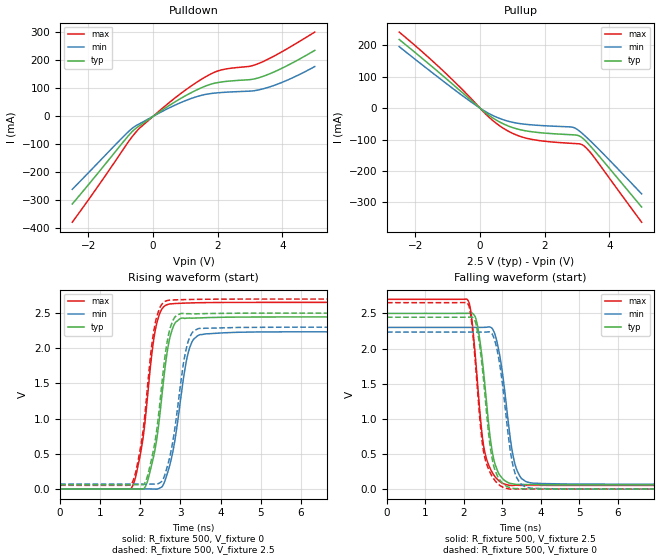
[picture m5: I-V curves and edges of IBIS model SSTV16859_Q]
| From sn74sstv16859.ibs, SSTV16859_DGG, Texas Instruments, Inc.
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[Model]   SSTV16859_Q
Model_type  Output
Vref =   1.25
Rref =   50
Cref =   30p
Vmeas =   1.25
| variable   typ   min   max
C_comp   5.86pF   1.92pF   9.72pF
| C_pullup   7.12pF   1.92pF   9.72pF
| C_pulldown   4.59pF   2.89pF   7.94pF
[Temperature Range]   40   85   0
| Ambient temperature   25   70   0
[Voltage range]   2.5   2.3   2.7
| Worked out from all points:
|   slope of the pulldown table from 0 to 0.375 V, typ, clamps not added: 12.7 ohm
|   slope of the pullup table from 0 to 0.375 V, typ, clamps not added: 12.6 ohm
|   rising waveform, R_fixture 500, V_fixture 0: 20-80 % time 331ps typ, 358ps min, 321ps max; typ from 0 V to 2.44 V
|   falling waveform, R_fixture 500, V_fixture 2.5: 20-80 % time 293ps typ, 319ps min, 272ps max; typ from 2.5 V to 0.06 V
|   rising waveform, R_fixture 500, V_fixture 2.5: 20-80 % time 320ps typ, 340ps min, 313ps max; typ from 0.06 V to 2.5 V
|   falling waveform, R_fixture 500, V_fixture 0: 20-80 % time 286ps typ, 308ps min, 265ps max; typ from 2.44 V to 0 V
[Pulldown]
| SSTV16859_Q
|   Voltage   I(typ)   I(min)   I(max)
-2.5V     -313.2mA   -260.7mA   -378.3mA
-910mV    -89.51mA   -71.28mA   -115.6mA
-550mV    -44.37mA   -34.85mA   -58.82mA
-360mV    -28.68mA   -22.72mA   -36.14mA
700mV     53.31mA    41.25mA    67.71mA
1.38V     96.13mA    71.48mA    124.1mA
1.92V     119mA      83.27mA    158.7mA
2.28V     125.2mA    86.44mA    169.8mA
3.02V     131.7mA    90.39mA    179.8mA
3.44V     144.6mA    99.57mA    197.8mA
4.14V     180.8mA    128.9mA    241.2mA
5V        235.7mA    177.9mA    301.2mA
[Pullup]
| SSTV16859_Q
|   Voltage   I(typ)   I(min)   I(max)
-2.5V     218.3mA    195.6mA    241.8mA
-1.265V   113.1mA    95.84mA    130.6mA
-165mV    15.03mA    11.66mA    18.54mA
305mV     -24.89mA   -18.76mA   -31.42mA
750mV     -51.43mA   -38.03mA   -65.87mA
1.13V     -65.79mA   -47.58mA   -85.66mA
1.525V    -74.13mA   -52.67mA   -97.93mA
2.85V     -84.82mA   -60.61mA   -112.3mA
3.055V    -87.94mA   -71.4mA    -113.6mA
3.22V     -99.68mA   -85.74mA   -120.6mA
3.51V     -132mA     -114mA     -153.5mA
5V        -314.6mA   -273mA     -363mA
[Ramp]
| SSTV16859_Q
| variable   typ   min   max
dV/dt_r   1.47/3.32E-10   1.34/3.64E-10   1.59/3.26E-10
dV/dt_f   1.47/2.94E-10   1.34/3.25E-10   1.59/2.77E-10
R_load = 500
[Rising Waveform]
| SSTV16859_Q
R_fixture =   500
C_fixture =   0
L_fixture =   0
V_fixture =   0
V_fixture_min = 0
V_fixture_max = 0
|   Time   V(typ)   V(min)   V(max)
0s        1.619nV    1.929nV    2.776nV
1.785ns   15.8uV     620.4nV    20.49mV
2.04ns    -1.588mV   -7.035uV   623mV
2.205ns   165mV      -41.87uV   1.474V
2.415ns   734.8mV    -1.963mV   2.37V
2.745ns   2.172V     365.9mV    2.632V
2.89ns    2.377V     798.7mV    2.638V
3.205ns   2.43V      1.962V     2.644V
3.64ns    2.436V     2.206V     2.65V
40ns      2.445V     2.234V     2.653V
[Falling Waveform]
| SSTV16859_Q
R_fixture =   500
C_fixture =   0
L_fixture =   0
V_fixture =   2.5
V_fixture_min = 2.3
V_fixture_max = 2.7
|   Time   V(typ)   V(min)   V(max)
0s        2.5V       2.3V       2.7V
2.1ns     2.501V     2.3V       2.69V
2.33ns    2.385V     2.3V       1.68V
2.555ns   1.432V     2.302V     499.1mV
2.79ns    394.2mV    2.228V     191.7mV
2.975ns   169.8mV    1.759V     91.65mV
3.2ns     81.95mV    750.9mV    52.3mV
3.47ns    66.57mV    171mV      52.44mV
4.025ns   62.02mV    78.47mV    52.56mV
40ns      60.39mV    69.99mV    51.99mV
[Rising Waveform]
| SSTV16859_Q
R_fixture =   500
C_fixture =   0
L_fixture =   0
V_fixture =   2.5
V_fixture_min = 2.3
V_fixture_max = 2.7
|   Time   V(typ)   V(min)   V(max)
0s        60.39mV    69.99mV    51.99mV
1.78ns    60.39mV    69.99mV    69.23mV
2.025ns   59.49mV    69.98mV    661.8mV
2.2ns     229.5mV    69.97mV    1.59V
2.405ns   826mV      67.9mV     2.442V
2.61ns    1.869V     201.6mV    2.666V
2.73ns    2.261V     448.6mV    2.685V
3.15ns    2.492V     2.009V     2.693V
3.48ns    2.492V     2.283V     2.697V
40ns      2.5V       2.3V       2.7V
[Falling Waveform]
| SSTV16859_Q
R_fixture =   500
C_fixture =   0
L_fixture =   0
V_fixture =   0
V_fixture_min = 0
V_fixture_max = 0
|   Time   V(typ)   V(min)   V(max)
0s        2.445V     2.234V     2.653V
2.095ns   2.446V     2.234V     2.644V
2.195ns   2.448V     2.234V     2.404V
2.325ns   2.326V     2.234V     1.615V
2.535ns   1.416V     2.234V     468.9mV
2.78ns    319.8mV    2.153V     142.3mV
3.195ns   21.62mV    591.6mV    295.3uV
3.385ns   7.028mV    152.5mV    2.083mV
3.815ns   2.38mV     9.737mV    1.004mV
40ns      419.9pV    4.133nV    3.556nV
